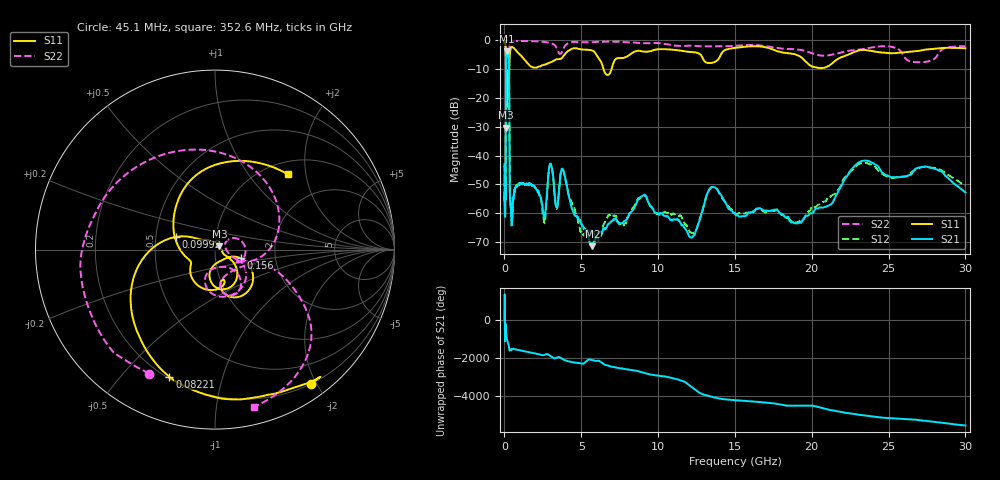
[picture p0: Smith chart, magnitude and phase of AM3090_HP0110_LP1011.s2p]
! Date/Time: Thu, Feb 28, 2019 2:00 PM
! Network Analyzer: Agilent Technologies E8364B Rev: A.07.50.67
! Sweep from 0.010 to 30.000 GHz, 1601 Points, Sweep Type: LOG
! Power Supply: 5.023 V, 0.002 A
# Hz S DB R 50
!freq MagS11 AngS11 MagS21 AngS21 MagS12 AngS12 MagS22 AngS22
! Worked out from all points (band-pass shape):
!   1601 points, 10 MHz to 30 GHz, reference 50 ohm
!   highest |S21| = -3.92 dB at 164.8 MHz (marker M1); lowest = -71.4 dB at 5.725 GHz (marker M2)
!   |S21| within 3 dB of the highest: 111.6 MHz to 285.1 MHz (173.5 MHz wide, 87.5 % of centre)
!   lowest |S11| = -30.3 dB at 107.7 MHz (marker M3), VSWR 1.06, Z = 52.5 + j1.85 ohm
!   |S11| at or under -10 dB: 98.38 MHz to 314.3 MHz (215.9 MHz wide, 105 % of centre); 6.446 GHz to 6.977 GHz (530.9 MHz wide, 7.91 % of centre)
!   |S22| runs from -24.7 to -0.2 dB; largest |S21 - S12| = 0.013
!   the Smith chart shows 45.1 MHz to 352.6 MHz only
!   S11 on the Smith chart (normalised r, x): 45.1 MHz: 0.20, -1.93; 82.21 MHz: 0.21, -0.68; 99.92 MHz: 0.63, +0.09; 156 MHz: 1.32, -0.13; 352.6 MHz: 1.24, +1.58
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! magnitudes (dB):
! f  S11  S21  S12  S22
! 10 MHz  -0.3  -42.9  -43.8  -0.7
! 38.04 MHz  -0.5  -58.9  -58.0  -1.6
! 45.1 MHz  -0.7  -57.4  -54.3  -2.1
! 82.21 MHz  -2.5  -51.6  -51.3  -4.7
! 99.92 MHz  -12.8  -16.1  -16.1  -12.2
! 107.7 MHz  -30.3  -8.3  -8.3  -24.2
! 123.3 MHz  -12.9  -5.3  -5.3  -16.1
! 144.7 MHz  -23.1  -4.2  -4.1  -17.7
! 156 MHz  -16.5  -4.0  -3.9  -16.3
! 164.8 MHz  -12.5  -3.9  -3.9  -13.9
! 290.1 MHz  -15.4  -7.7  -7.6  -15.1
! 352.6 MHz  -4.7  -53.1  -52.3  -0.9
! 550.5 MHz  -2.6  -56.3  -56.7  -0.3
! 2.084 GHz  -9.6  -51.7  -51.7  -0.5
! 2.584 GHz  -8.5  -60.8  -63.0  -0.7
! 2.958 GHz  -7.8  -43.2  -43.1  -1.0
! 3.385 GHz  -6.7  -57.9  -58.5  -2.7
! 3.817 GHz  -5.7  -45.0  -45.1  -3.3
! 5.725 GHz  -3.7  -71.4  -67.2  -0.8
! 7.926 GHz  -5.9  -62.2  -63.5  -0.8
! 23.48 GHz  -3.5  -41.8  -42.6  -3.0
! 30 GHz  -2.9  -52.8  -50.4  -2.1
